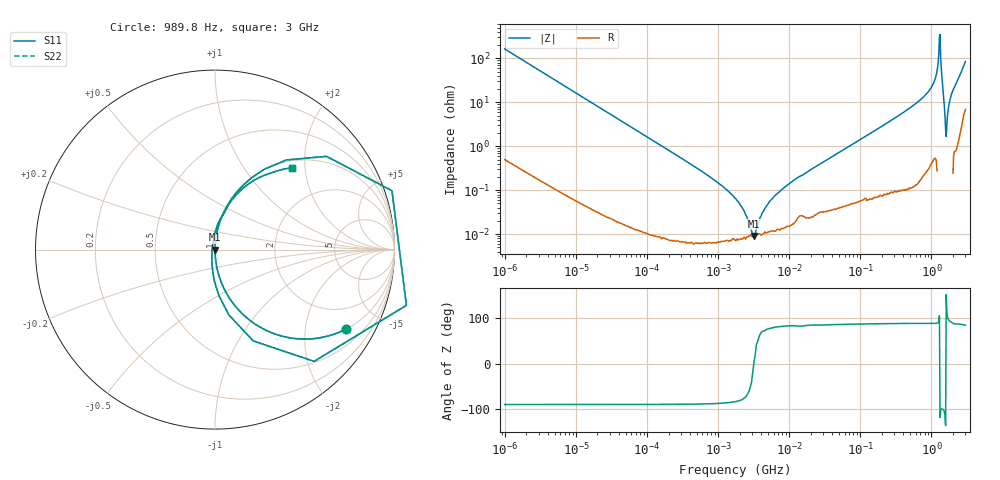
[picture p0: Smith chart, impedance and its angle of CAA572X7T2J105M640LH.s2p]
! S-Parameter Data Generated by TDK Corporation
! Copyright(C) 2020 TDK Corporation.
! All Rights Reserved.
! TDK P/N: CAA572X7T2J105M640LH (Multilayer Ceramic Chip Capacitor)
! Property: C=1uF
! Size(LxWxT): 6x5x6.4mm
! Model Type: s2p (Touchstone File Format Version 1.0)
! Frequency: DC=Yes Start=0.000989846MHz Stop=3000MHz 463points Log-sweep
! Model Generated on Nov. 18, 2020
! Port Assignments:
!  1 ---| |--- 2
! Applicable Conditions:
!  Temperature = 25 degC
!  DC Bias Voltage = 0 V
!  Small Signal Operation
! Terms and conditions regarding TDK Simulation Models
! (1)This simulation model is being provided solely for informational purposes. Please refer to the specifications of the products in terms of detailed characteristics of such products.
! (2)In no event shall TDK Corporation of any of its subsidiaries be liable for any loss or damage arising, directly or indirectly,
!  From any information contained in this simulation model, including, but not limited to loss or damages arising from any inaccuracies, omissions or errors in connection with such information.
! (3)Any and all copyrights on this simulation model are owned by TDK Corporation.
!  Duplication or redistribution of this simulation model without prior written permission from TDK Corporation is prohibited.
! (4)This simulation model is subject to any modification or change without any prior notice.
! (5)Neither TDK Corporation nor any of its subsidiaries shall make any warranty, express or implied,
!  Including but not limited to the correctness, implied warranties of merchantability and fitness for a particular purpose with respect to this simulation models.
! (6)The use of this simulation model shall be deemed to have consented to the terms and conditions hereof.
# Hz S MA R 50
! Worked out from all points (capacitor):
!   462 points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, 989.8 Hz to 3 GHz, reference 50 ohm
!   read as one part in series: C = 979 nF near 1.07 kHz
!   lowest |Z| = 9.13 mohm at 3.186 MHz (marker M1)
!   series resonance near 3.163 MHz, so ESL is about 2.6 nH
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989.846  0.8529 -31.3  0.5195 58.5  0.5195 58.5  0.8529 -31.3
3587.28  0.413 -65.4  0.9094 24.4  0.9094 24.4  0.413 -65.4
12024.64  0.1345 -82.1  0.9904 7.7  0.9904 7.7  0.1345 -82.1
146075.1  0.01121 -88.9  0.9999 0.6  0.9999 0.6  0.01121 -88.9
1774518  0.0006377 -83.5  0.9999 0.0  0.9999 0.0  0.0006377 -83.5
3186112  9.132e-05 4.1  0.9999 -0.0  0.9999 -0.0  9.132e-05 4.1
5720602  0.0006365 79.2  0.9999 -0.0  0.9999 -0.0  0.0006365 79.2
2.073191e7  0.00304 85.2  0.9997 -0.2  0.9997 -0.2  0.00304 85.2
2.507343e8  0.03585 86.6  0.9985 -2.1  0.9985 -2.1  0.03585 86.6
6.821091e8  0.11 82.8  0.9923 -6.3  0.9923 -6.3  0.11 82.8
1.059487e9  0.2547 74.2  0.9625 -14.8  0.9625 -14.8  0.2547 74.2
1.171007e9  0.3934 66.2  0.9152 -23.2  0.9152 -23.2  0.3934 66.2
1.243477e9  0.6384 51.5  0.7826 -39.7  0.7826 -39.7  0.6384 51.5
1.294266e9  1.039 18.4  0.3282 -87.6  0.3282 -87.6  1.039 18.4
1.374365e9  0.5515 -67.3  0.937 32.9  0.937 32.9  0.5515 -67.3
1.430499e9  0.258 -85.1  1.011 14.7  1.011 14.7  0.258 -85.1
1.54974e9  0.0489 -111.1  1.019 2.6  1.019 2.6  0.0489 -111.1
1.613037e9  0.01693 152.4  1.015 -0.4  1.015 -0.4  0.01693 152.4
1.782824e9  0.09841 89.2  1.003 -5.6  1.003 -5.6  0.09841 89.2
1.931433e9  0.1576 82.0  0.9905 -9.1  0.9905 -9.1  0.1576 82.0
2.455801e9  0.3529 67.0  0.9215 -20.6  0.9215 -20.6  0.3529 67.0
3e9  0.6248 46.9  0.732 -38.5  0.732 -38.5  0.6248 46.9
